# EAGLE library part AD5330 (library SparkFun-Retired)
8-bit parallel input DAC Retired: IC-09612
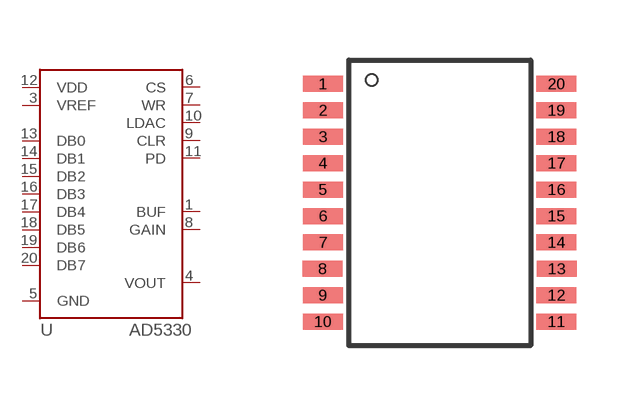
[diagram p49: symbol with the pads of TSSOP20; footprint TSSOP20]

Designator prefix U

## AD5330  [TSSOP20]
1  BUF
3  VREF
4  VOUT
5  GND
6  CS
7  WR
8  GAIN
9  CLR
10  LDAC
11  PD
12  VDD
13  DB0
14  DB1
15  DB2
16  DB3
17  DB4
18  DB5
19  DB6
20  DB7

## Footprint TSSOP20 (pad centres in mm)
smd 1 x 0.4: 1 -2.937,2.693; 2 -2.937,2.032; 3 -2.937,1.372; 4 -2.937,0.712; 5 -2.937,0.051; 6 -2.937,-0.609; 7 -2.937,-1.27; 8 -2.943,-1.93; 9 -2.937,-2.59; 10 -2.937,-3.251; 11 2.905,-3.251; 12 2.905,-2.59; 13 2.911,-1.93; 14 2.905,-1.27; 15 2.905,-0.609; 16 2.905,0.051; 17 2.905,0.712; 18 2.905,1.372; 19 2.905,2.032; 20 2.905,2.693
